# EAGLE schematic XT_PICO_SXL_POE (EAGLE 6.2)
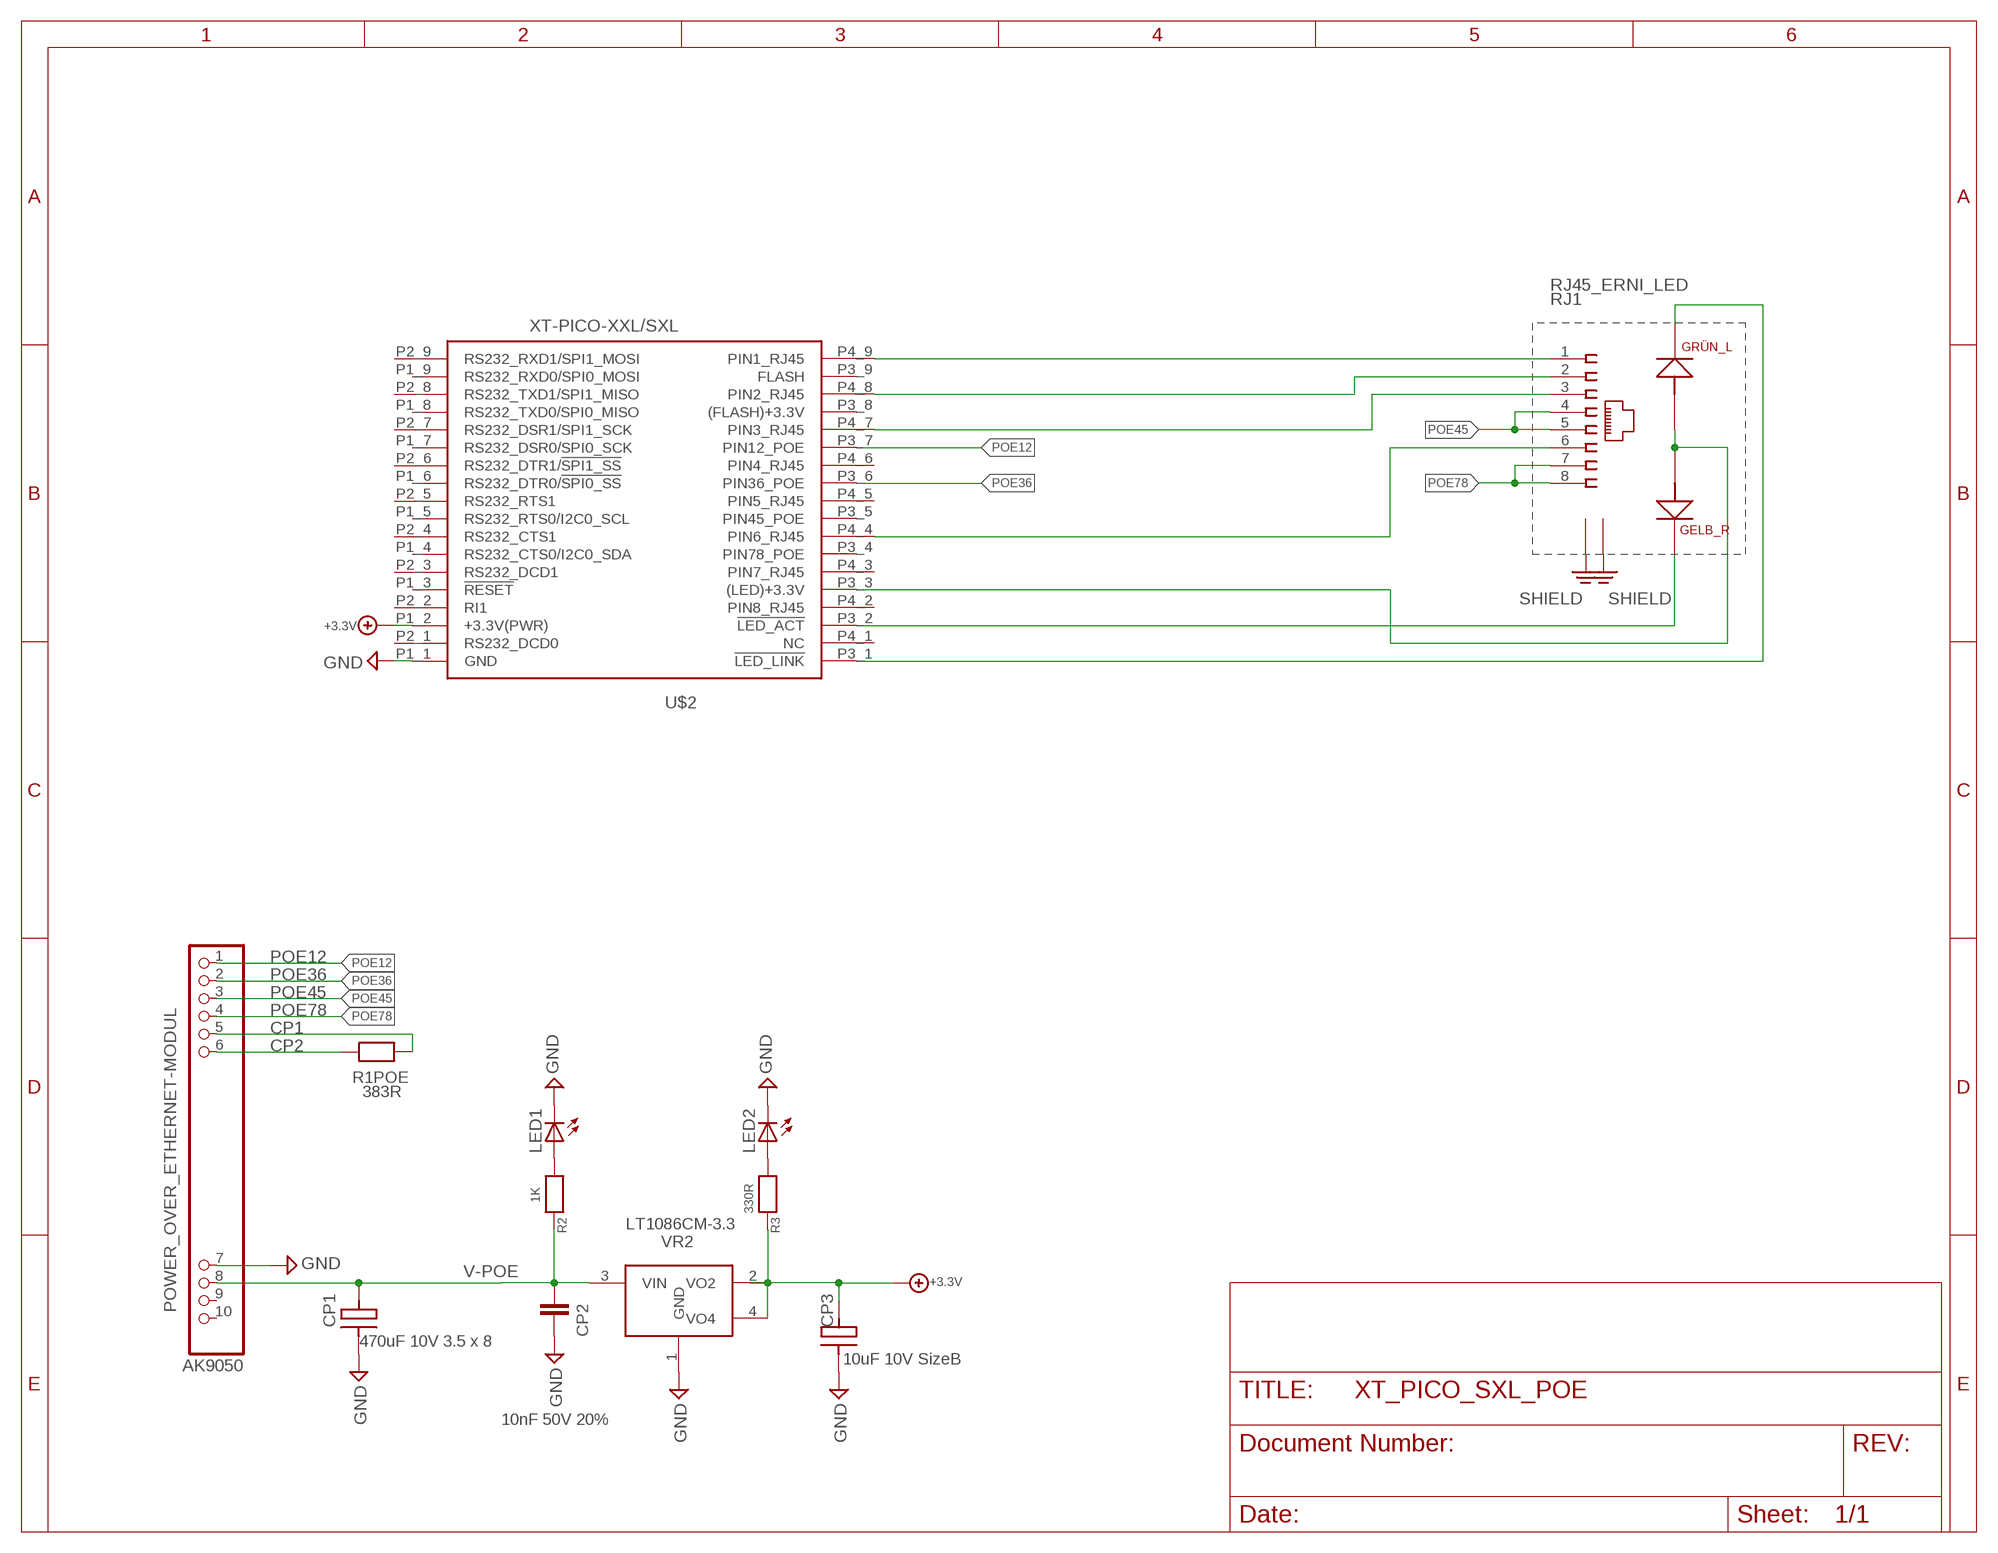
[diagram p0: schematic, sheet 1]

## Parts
CP1  470uF 10V 3.5 x 8  C3528_B  [ORCAD_X_CT3528]
CP2  10nF 50V 20%  CHIP-C-0603  [SMD-0603]
CP3  10uF 10V SizeB  C3528_B  [ORCAD_X_CT3528]
LED1  LED3MM  [LED3MM]
LED2  LED3MM  [LED3MM]
POWER_OVER_ETHERNET-MODUL  AK9050  POE_AG9000  [POE_AG9000]
R1POE  383R  CHIP-R-0603  [SMD-0603]
R2  1K  CHIP-R-0603  [SMD-0603]
R3  330R  CHIP-R-0603  [SMD-0603]
RJ1  RJ45_ERNI_LED  [ORCAD_X_ERNI_RJ45_LED]
U$2  XT-PICO-XXL/SXL  [XT-PICO-XXL/SXL]
VR2  LT1086CM-3.3  LT1086_5.0  [DPAK_223]

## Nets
+3.3V: CP3.1(C+) R3.2 U$2.P1_2(+3.3V(PWR)) VR2.2(VO2) VR2.4(VO4)
CP1: POWER_OVER_ETHERNET-MODUL.5(CP1) R1POE.1
CP2: POWER_OVER_ETHERNET-MODUL.6(CP2) R1POE.2
GND: CP1.2(C-) CP2.1 CP3.2(C-) LED1.K(C) LED2.K(C) POWER_OVER_ETHERNET-MODUL.7(GND) U$2.P1_1(GND) VR2.1(GND)
N$1: CP2.2 R2.2 VR2.3(VIN)
N$7: RJ1.1 U$2.P4_9(PIN1_RJ45)
N$8: RJ1.2 U$2.P4_8(PIN2_RJ45)
N$9: RJ1.3 U$2.P4_7(PIN3_RJ45)
N$12: RJ1.6 U$2.P4_4(PIN6_RJ45)
N$15: RJ1.A1 RJ1.A2 U$2.P3_3((LED)+3.3V)
N$16: RJ1.K1 U$2.P3_2(!LED_ACT)
N$17: RJ1.K2 U$2.P3_1(!LED_LINK)
N$37: LED1.A R2.1
N$38: LED2.A R3.1
PE: RJ1.9 RJ1.10 ; supply symbol labelled SHIELD
POE12: POWER_OVER_ETHERNET-MODUL.1(VA1) U$2.P3_7(PIN12_POE)
POE36: POWER_OVER_ETHERNET-MODUL.2(VA2) U$2.P3_6(PIN36_POE)
POE45: POWER_OVER_ETHERNET-MODUL.3(VB1) RJ1.4 RJ1.5
POE78: POWER_OVER_ETHERNET-MODUL.4(VB2) RJ1.7 RJ1.8
V-POE: CP1.1(C+) POWER_OVER_ETHERNET-MODUL.8(VDC+)
Unconnected: POWER_OVER_ETHERNET-MODUL.9(ADJ) POWER_OVER_ETHERNET-MODUL.10(IC) U$2.P1_3(!RESET) U$2.P1_4(RS232_CTS0/I2C0_SDA) U$2.P1_5(RS232_RTS0/I2C0_SCL) U$2.P1_6(RS232_DTR0/!SPI0_SS!) U$2.P1_7(RS232_DSR0/SPI0_SCK) U$2.P1_8(RS232_TXD0/SPI0_MISO) U$2.P1_9(RS232_RXD0/SPI0_MOSI) U$2.P2_1(RS232_DCD0) U$2.P2_2(RI1) U$2.P2_3(RS232_DCD1) U$2.P2_4(RS232_CTS1) U$2.P2_5(RS232_RTS1) U$2.P2_6(RS232_DTR1/!SPI1_SS!) U$2.P2_7(RS232_DSR1/SPI1_SCK) U$2.P2_8(RS232_TXD1/SPI1_MISO) U$2.P2_9(RS232_RXD1/SPI1_MOSI) U$2.P3_4(PIN78_POE) U$2.P3_5(PIN45_POE) U$2.P3_8((FLASH)+3.3V) U$2.P3_9(FLASH) U$2.P4_1(NC) U$2.P4_2(PIN8_RJ45) U$2.P4_3(PIN7_RJ45) U$2.P4_5(PIN5_RJ45) U$2.P4_6(PIN4_RJ45)

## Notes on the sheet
- 10nF 50V 20%

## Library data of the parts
CP1 CP3 = XTMACRO_AS:C3528_B
CP2 = mea-lib:CHIP-C-?: Chip capacitance
LED1 LED2 = led:LED: LED
POWER_OVER_ETHERNET-MODUL = XTMACRO:POE_AG9000: PIN HEADER
R1POE = mea-lib:CHIP-R-?: Chip resistors
R2 R3 = XTMACRO:CHIP-R-?: Chip resistors
RJ1 = XTMACRO:RJ45_ERNI_LED
U$2 = ak-devices:XT-PICO-XXL/SXL: AK-NORD XT-PICO-XXL/SXL
VR2 = XTMACRO_AS:LT1086_5.0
